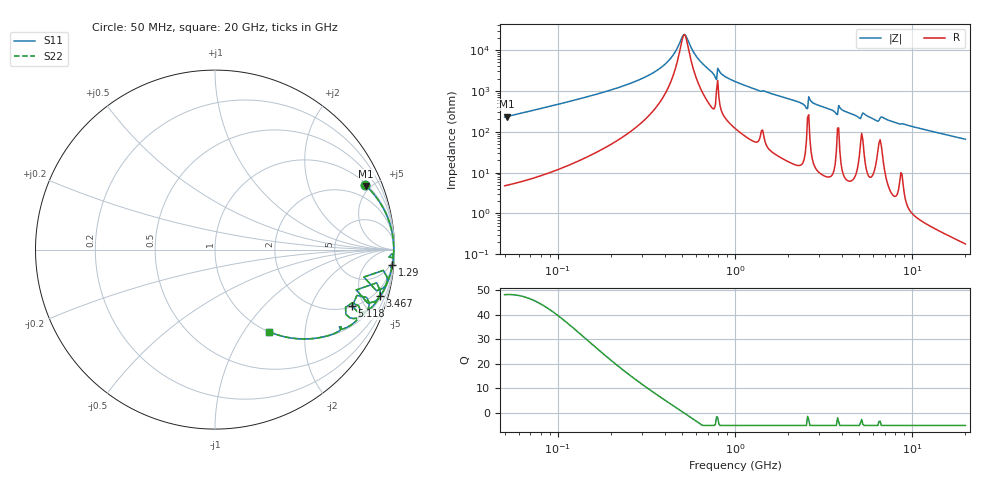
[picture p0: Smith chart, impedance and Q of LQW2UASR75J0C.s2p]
!Murata Part Number: LQW2UASR75J0C
!These Parameters are Measured in Series Mode Connection
!  o--[Z]--o
!Port1  Port2
!  o-------o
!Freq. Start=50[MHz] Stop=20[GHz], 401[Steps]
# Hz S RI R 50
!Freq.(Hz) S11(Real) S11(Imag) S21(Real) S21(Imag) S12(Real) S12(Imag) S22(Real) S22(Imag)
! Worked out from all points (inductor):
!   401 points, 50 MHz to 20 GHz, reference 50 ohm
!   read as one part in series: L = 720 nH near 51.52 MHz
!   highest Q = 48.1 at 51.52 MHz (marker M1), where L = 727 nH
!   self-resonance near 517.3 MHz
!   S11 on the Smith chart (normalised r, x): 50 MHz: 1.10, +4.57; 1.29 GHz: 2, -22; 3.467 GHz: 1.16, -7.01; 5.118 GHz: 2.05, -4.07; 20 GHz: 1.00, -1.31
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5e7  0.8341 0.3618  0.1659 -0.3618  0.1659 -0.3618  0.8341 0.3618
5.152053e7  0.8421 0.3544  0.1579 -0.3544  0.1579 -0.3544  0.8421 0.3544
1.364002e8  0.9733 0.1462  0.0267 -0.1462  0.0267 -0.1462  0.9733 0.1462
2.558771e8  0.9915 0.0646  0.00848 -0.0646  0.00848 -0.0646  0.9915 0.0646
3.721004e8  0.995 0.0286  0.00499 -0.0286  0.00499 -0.0286  0.995 0.0286
4.387496e8  0.9957 0.0142  0.00435 -0.0142  0.00435 -0.0142  0.9957 0.0142
5.173368e8  0.9959 3.32e-05  0.00414 -3.32e-05  0.00414 -3.32e-05  0.9959 3.32e-05
6.100003e8  0.9956 -0.0143  0.00436 0.0143  0.00436 0.0143  0.9956 -0.0143
7.636728e8  0.9923 -0.04  0.00774 0.04  0.00774 0.04  0.9923 -0.04
8.230629e8  0.9935 -0.0342  0.00654 0.0342  0.00654 0.0342  0.9935 -0.0342
1e9  0.9924 -0.058  0.00758 0.058  0.00758 0.058  0.9924 -0.058
1.289994e9  0.9876 -0.0879  0.0124 0.0879  0.0124 0.0879  0.9876 -0.0879
2.493527e9  0.933 -0.217  0.067 0.217  0.067 0.217  0.933 -0.217
2.728004e9  0.958 -0.1807  0.042 0.1807  0.042 0.1807  0.958 -0.1807
3.466789e9  0.9197 -0.2606  0.0803 0.2606  0.0803 0.2606  0.9197 -0.2606
3.680849e9  0.8863 -0.2911  0.1137 0.2911  0.1137 0.2911  0.8863 -0.2911
3.967106e9  0.9183 -0.2514  0.0817 0.2514  0.0817 0.2514  0.9183 -0.2514
5.117541e9  0.7642 -0.3147  0.2358 0.3147  0.2358 0.3147  0.7642 -0.3147
6.701223e9  0.7991 -0.3121  0.2009 0.3121  0.2009 0.3121  0.7991 -0.3121
7.442007e9  0.7747 -0.4073  0.2253 0.4073  0.2253 0.4073  0.7747 -0.4073
1.201863e10  0.5489 -0.4951  0.4511 0.4951  0.4511 0.4951  0.5489 -0.4951
2e10  0.301 -0.4573  0.699 0.4573  0.699 0.4573  0.301 -0.4573
